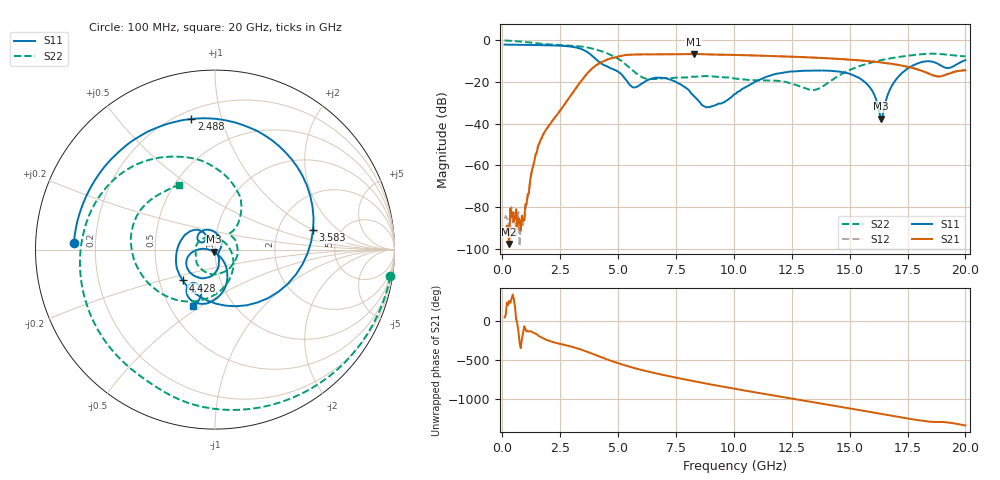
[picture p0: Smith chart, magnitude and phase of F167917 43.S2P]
!  2-Port S-parameters saved by WinCal
! VAR MeasName=S-Parameters (CALIBRATED_DATA) read from VNA (N5242A)
! VAR MeasDate=2016-11-22 9:01:54
! VAR NAME=F167917 43
! VAR FILENAME=F167917 43.S2P
! VAR DATE=2016-11-22 9:01:54
! VAR PHYS_PORTS=1,2
# Hz S DB R 50
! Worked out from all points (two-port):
!   401 points, 100 MHz to 20 GHz, reference 50 ohm
!   highest |S21| = -6.56 dB at 8.259 GHz (marker M1); lowest = -97.6 dB at 299 MHz (marker M2)
!   |S21| within 3 dB of the highest: 4.479 GHz to 15.37 GHz (10.9 GHz wide, 110 % of centre)
!   lowest |S11| = -37.5 dB at 16.37 GHz (marker M3), VSWR 1.03, Z = 49.3 - j1.13 ohm
!   |S11| at or under -10 dB: 4.136 GHz to 19.89 GHz (15.76 GHz wide, 131 % of centre)
!   |S22| runs from -23.9 to -0.1 dB; largest |S21 - S12| = 0.0049
!   S11 on the Smith chart (normalised r, x): 100 MHz: 0.12, +0.02; 2.488 GHz: 0.25, +0.80; 3.583 GHz: 3.17, +1.01; 4.428 GHz: 0.66, -0.24; 20 GHz: 0.66, -0.46
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1e8  -2.09 177.3  -91.59 43.8  -85.47 72.1  -0.10 -8.7
2.99e8  -2.11 172.0  -97.62 -103.3  -89.86 62.8  -0.23 -25.0
9.955e8  -2.22 153.3  -78.62 -98.6  -82.69 -126.7  -0.83 -77.5
1.64225e9  -2.34 134.0  -47.97 156.7  -47.94 155.9  -1.69 -117.5
2.488e9  -2.62 100.3  -33.91 66.2  -33.87 66.1  -2.23 -160.4
3.43325e9  -4.30 29.5  -19.11 -10.5  -19.13 -10.4  -3.04 153.1
3.5825e9  -5.08 11.3  -17.02 -26.2  -17.02 -26.1  -3.28 145.4
3.9805e9  -8.44 -51.0  -12.59 -72.9  -12.55 -72.8  -4.26 124.4
4.42825e9  -12.06 -136.5  -9.76 -123.9  -9.71 -124.2  -5.79 101.3
5.274e9  -18.05 125.2  -7.15 152.2  -7.15 152.0  -11.09 57.9
5.72175e9  -22.63 141.7  -6.84 112.9  -6.84 112.9  -15.28 46.9
6.7665e9  -17.93 130.1  -6.74 38.0  -6.75 37.8  -18.50 39.1
8.259e9  -26.62 40.5  -6.56 -53.4  -6.59 -53.3  -17.48 -62.0
8.90575e9  -32.06 -22.7  -6.77 -90.7  -6.78 -90.7  -17.23 -103.9
1.005e10  -25.73 -67.1  -7.02 -152.4  -7.03 -152.2  -18.36 -150.1
1.1841e10  -16.05 -102.4  -7.67 115.1  -7.62 115.4  -19.40 169.1
1.338325e10  -14.53 -133.3  -8.28 37.6  -8.22 37.6  -23.84 62.5
1.547275e10  -18.50 -175.6  -9.67 -67.9  -9.69 -68.4  -12.20 -88.0
1.636825e10  -37.51 -120.8  -10.66 -114.6  -10.67 -114.0  -9.52 -120.5
1.67165e10  -24.22 -53.3  -11.11 -132.4  -11.18 -131.9  -8.75 -132.1
1.786075e10  -11.43 -87.1  -13.74 169.4  -13.63 169.8  -6.95 -170.1
2e10  -9.50 -111.3  -14.39 97.0  -14.24 96.7  -7.71 118.8
